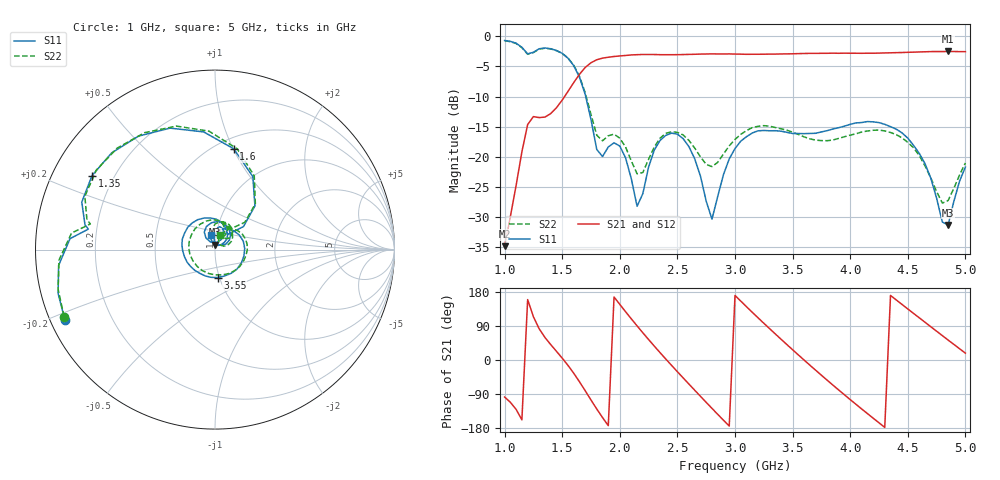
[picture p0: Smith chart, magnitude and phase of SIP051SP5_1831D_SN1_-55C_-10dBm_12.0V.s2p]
# GHz  S  dB  R  50
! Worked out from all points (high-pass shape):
!   81 points, 1 GHz to 5 GHz, reference 50 ohm
!   highest |S21| = -2.52 dB at 4.85 GHz (marker M1); lowest = -34.8 dB at 1 GHz (marker M2)
!   |S21| within 3 dB of the highest: 1.684 GHz to end of sweep
!   lowest |S11| = -31.3 dB at 4.85 GHz (marker M3), VSWR 1.06, Z = 49.9 + j2.72 ohm
!   |S11| at or under -10 dB: 1.704 GHz to end of sweep
!   |S22| runs from -27.7 to -0.7 dB; largest |S21 - S12| = 0.0023
!   S11 on the Smith chart (normalised r, x): 1 GHz: 0.04, -0.22; 1.35 GHz: 0.12, +0.27; 1.6 GHz: 0.60, +1.01; 3.55 GHz: 0.98, -0.31; 5 GHz: 0.94, +0.15
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1  -0.69 -155.0  -34.80 -97.7  -34.80 -96.8  -0.73 -156.1
1.2  -2.92 170.8  -14.64 159.4  -14.65 159.5  -2.98 168.4
1.35  -1.94 148.9  -13.39 59.5  -13.37 59.6  -1.98 146.2
1.5  -2.83 110.3  -10.58 4.9  -10.58 4.9  -2.84 107.4
1.6  -4.87 79.4  -7.67 -34.9  -7.66 -35.0  -4.80 77.6
1.7  -9.64 47.5  -5.16 -81.3  -5.17 -81.3  -9.37 48.6
1.8  -18.76 49.1  -3.89 -129.3  -3.90 -129.3  -16.39 51.5
1.95  -17.66 77.7  -3.35 166.3  -3.36 166.4  -16.22 68.2
2.15  -28.18 80.4  -3.05 90.0  -3.04 90.1  -22.80 67.1
2.35  -17.25 110.5  -3.05 19.2  -3.04 19.2  -16.87 89.6
2.5  -16.22 70.8  -3.05 -30.9  -3.04 -30.9  -15.92 60.9
2.7  -23.17 27.0  -2.95 -95.8  -2.94 -95.8  -19.99 39.4
2.8  -30.32 69.1  -2.92 -127.6  -2.91 -127.6  -21.61 53.2
3  -18.61 72.9  -2.95 170.4  -2.95 170.4  -17.10 55.4
3.25  -15.62 2.3  -2.97 97.0  -2.97 97.0  -14.82 9.9
3.55  -16.12 -84.7  -2.87 13.4  -2.88 13.3  -16.28 -60.4
3.7  -16.08 -122.2  -2.84 -26.9  -2.83 -26.9  -17.21 -104.8
4  -14.60 172.0  -2.81 -104.5  -2.82 -104.4  -16.38 161.0
4.35  -14.98 98.6  -2.74 170.3  -2.75 170.3  -15.95 73.8
4.6  -19.42 49.0  -2.60 111.2  -2.59 111.2  -19.77 27.0
4.85  -31.29 90.4  -2.52 52.6  -2.52 52.7  -27.22 56.4
5  -21.68 107.3  -2.55 18.1  -2.56 18.1  -21.01 69.9
